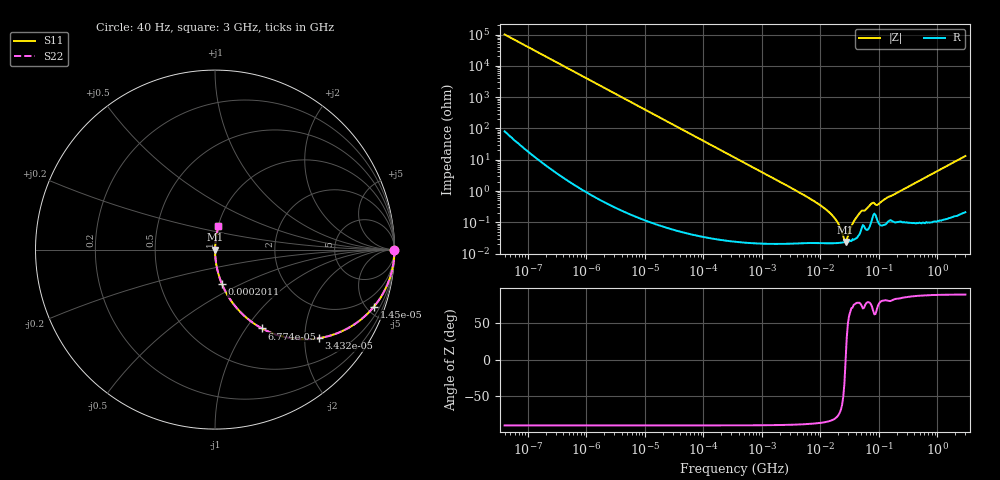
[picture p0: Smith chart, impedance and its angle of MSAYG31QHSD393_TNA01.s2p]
! MSAYG31QHSD393_TNA01  S-PARAMETER MODEL  ( General Type )
! Model Generated by TAIYO YUDEN Corporation (http://www.ty-top.com)
! Version 2.0
! TAIYO YUDEN Control No. 031016
! Copyright(c) 2003 TAIYO YUDEN CO.,LTD. All Rights Reserved.
! Product Description (link to TY-COMPAS)
! https://ds.yuden.co.jp/TYCOMPAS/or/detail?pn=MSAYG31QHSD393KTNA01&u=M
! Products Name : Multilayer Ceramic Capacitors
! Characteristics :
!  Capacitance : 0.039 uF , Rated Voltage : 35V
!  Case Size : 3.2 x 1.6 / 0.126 x 0.063 [mm/inch] , Thickness : 1.15 / 0.045 [mm/inch]
!  (Conditions: Temperature = 25 degC , DC Bias Current/Voltage = 0A / 0V)
! External Node Assignments :
!  1  o---| |---o  2
! GND o---------o GND
! Frequency Range : 40Hz  -  3GHz  [ 401 STEP ]
# MHz S RI R 50
! Freq[MHz].  S11 Real  S11 Imag  S21 Real  S21 Imag  S12 Real  S12 Imag  S22 Real  S22 Imag
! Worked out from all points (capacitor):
!   401 points, 40 Hz to 3 GHz, reference 50 ohm
!   read as one part in series: C = 39.4 nF near 44 Hz
!   lowest |Z| = 23.4 mohm at 26.89 MHz (marker M1)
!   series resonance near 26.92 MHz, so ESL is about 890 pH
!   S11 on the Smith chart (normalised r, x): 40 Hz: open; 14.5 kHz: 1.00, -5.57; 34.32 kHz: 1.00, -2.35; 67.74 kHz: 1.00, -1.19; 201.1 kHz: 1.00, -0.40; 3 GHz: 1.00, +0.26
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4e-05  1 -0.000991  1.77e-06 0.000991  1.77e-06 0.000991  1 -0.000991
0.000834  0.9996 -0.0207  0.000431 0.0207  0.000431 0.0207  0.9996 -0.0207
0.004265  0.9889 -0.1045  0.0111 0.1045  0.0111 0.1045  0.9889 -0.1045
0.014503  0.8856 -0.3182  0.1144 0.3182  0.1144 0.3182  0.8856 -0.3182
0.017386  0.8434 -0.3632  0.1566 0.3632  0.1566 0.3632  0.8434 -0.3632
0.034318  0.5804 -0.4933  0.4196 0.4933  0.4196 0.4933  0.5804 -0.4933
0.067738  0.2622 -0.4395  0.7378 0.4395  0.7378 0.4395  0.2622 -0.4395
0.111532  0.116 -0.3198  0.884 0.3198  0.884 0.3198  0.116 -0.3198
0.201066  0.039 -0.1929  0.961 0.1929  0.961 0.1929  0.039 -0.1929
0.362475  0.0125 -0.1099  0.9875 0.1099  0.9875 0.1099  0.0125 -0.1099
7.222098  0.000246 -0.00519  0.9998 0.00519  0.9998 0.00519  0.000246 -0.00519
16.33207  0.000217 -0.00158  0.9998 0.00158  0.9998 0.00158  0.000217 -0.00158
19.57906  0.000219 -0.000983  0.9998 0.000983  0.9998 0.000983  0.000219 -0.000983
24.56009  0.000228 -0.000275  0.9998 0.000275  0.9998 0.000275  0.000228 -0.000275
26.8909  0.000234 -2.79e-06  0.9998 2.79e-06  0.9998 2.79e-06  0.000234 -2.79e-06
29.4429  0.000241 0.000281  0.9998 -0.000281  0.9998 -0.000281  0.000241 0.000281
36.93337  0.000275 0.00101  0.9997 -0.00101  0.9997 -0.00101  0.000275 0.00101
48.47801  0.000507 0.00208  0.9995 -0.00208  0.9995 -0.00208  0.000507 0.00208
76.28187  0.00128 0.00391  0.9987 -0.00391  0.9987 -0.00391  0.00128 0.00391
95.68847  0.00107 0.00353  0.9989 -0.00353  0.9989 -0.00353  0.00107 0.00353
150.5692  0.00118 0.00656  0.9988 -0.00656  0.9988 -0.00656  0.00118 0.00656
3000  0.0191 0.1291  0.9809 -0.1291  0.9809 -0.1291  0.0191 0.1291
